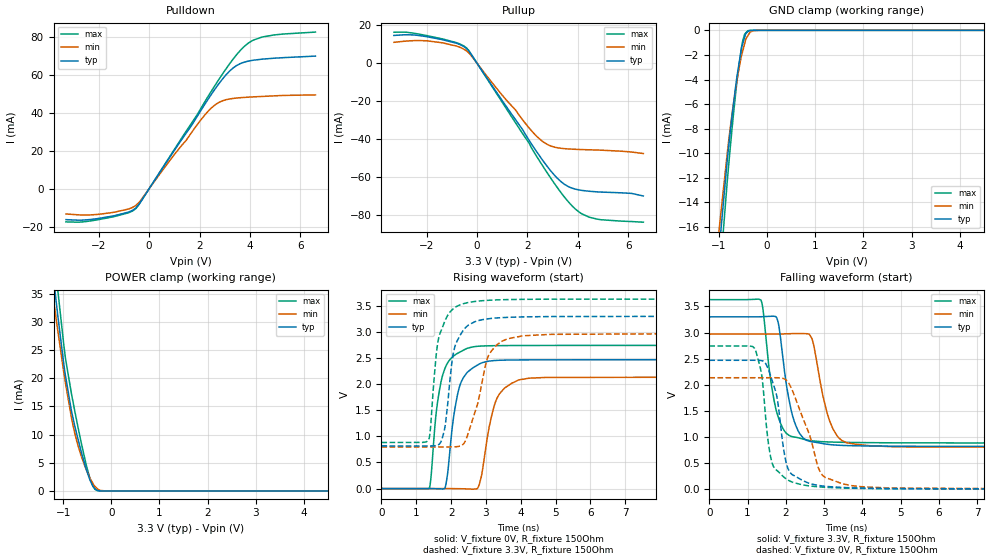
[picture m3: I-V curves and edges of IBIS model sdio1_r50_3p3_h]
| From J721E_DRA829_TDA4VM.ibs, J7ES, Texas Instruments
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|   r50_3p3_h
[Model]   sdio1_r50_3p3_h
Model_type   I/O
Polarity   Non-Inverting
Enable   Active-High
Vinl = 0
Vinh = 0.8
Vmeas = 1.65
Vref = 3.3
Cref = 2pF
Rref = 100000
|   typ   min   max
C_comp   2.899pF   2.635pF   3.167pF
[Voltage Range]   3.3   2.97   3.63
[Temperature Range]   27   150   -40
[Pullup Reference]   3.3   2.97   3.63
[Pulldown Reference]   0   0   0
[Power Clamp Reference]   3.3   2.97   3.63
[GND Clamp Reference]   0   0   0
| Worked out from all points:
|   slope of the pulldown table from 0 to 0.495 V, typ, clamps not added: 49.2 ohm
|   slope of the pullup table from 0 to 0.495 V, typ, clamps not added: 50.3 ohm
|   GND clamp passes 1 mA (typ) near -0.50 V on its own axis
|   POWER clamp passes 1 mA (typ) near -0.39 V on its own axis
|   falling waveform, V_fixture 3.3V, R_fixture 150Ohm: 20-80 % time 337ps typ, 401ps min, 323ps max; typ from 3.3 V to 0.817 V
|   rising waveform, V_fixture 0V, R_fixture 150Ohm: 20-80 % time 319ps typ, 386ps min, 306ps max; typ from 0 V to 2.47 V
|   rising waveform, V_fixture 3.3V, R_fixture 150Ohm: 20-80 % time 305ps typ, 492ps min, 309ps max; typ from 0.817 V to 3.3 V
|   falling waveform, V_fixture 0V, R_fixture 150Ohm: 20-80 % time 324ps typ, 574ps min, 258ps max; typ from 2.47 V to 0 V
[Pulldown]
|   Voltage   I(typ)   I(min)   I(max)
-3.3V     -16.37mA   -13.36mA   -17.55mA
-2.003V   -15.72mA   -13.55mA   -16.34mA
-825mV    -12.41mA   -10.77mA   -12.77mA
-528mV    -10.21mA   -8.836mA   -10.53mA
1.917V    38.43mA    33.99mA    39.31mA
2.363V    47.76mA    41.24mA    49.28mA
2.779V    55.67mA    45.65mA    57.95mA
3.184V    62.04mA    47.4mA     65.85mA
3.452V    64.93mA    47.89mA    70.52mA
3.937V    67.42mA    48.37mA    76.93mA
4.491V    68.47mA    48.75mA    80.18mA
6.6V      70.08mA    49.57mA    82.77mA
[GND Clamp]
|   Voltage   I(typ)   I(min)   I(max)
-3.3V     -160mA     -119.4mA   -217mA
-1.033V   -19.39mA   -17.52mA   -22.42mA
-825mV    -10.43mA   -9.877mA   -12.11mA
-716.1mV  -6.541mA   -6.437mA   -7.501mA
-627mV    -3.775mA   -4.073mA   -4.142mA
-537.9mV  -1.565mA   -2.149mA   -1.562mA
-508.2mV  -1.103mA   -1.7mA     -875.4uA
-468.6mV  -579.1uA   -1.102mA   -332.5uA
-399.3mV  -111.6uA   -431uA     -25.66uA
-349.8mV  -18.88uA   -131.7uA   -5.143uA
-171.6mV  -88.29nA   -2.802uA   -107.4nA
6.6V      0A         0A         0A
[Pullup]
|   Voltage   I(typ)   I(min)   I(max)
-3.3V     14.73mA    11.09mA    16.42mA
-1.993V   14.07mA    11.89mA    14.65mA
-825mV    10.65mA    9.143mA    10.95mA
-438.9mV  8.033mA    6.753mA    8.341mA
1.808V    -35.11mA   -29.93mA   -37.21mA
2.313V    -45.75mA   -37.91mA   -48.12mA
2.779V    -54.45mA   -42.85mA   -57.84mA
3.333V    -62.64mA   -44.97mA   -68.45mA
3.887V    -66.53mA   -45.51mA   -76.92mA
4.452V    -67.71mA   -45.77mA   -81.42mA
6.125V    -68.82mA   -46.93mA   -83.71mA
6.6V      -70.21mA   -47.75mA   -84.07mA
[POWER Clamp]
|   Voltage   I(typ)   I(min)   I(max)
-3.3V     224.5mA    191.3mA    262.6mA
-1.211V   38.57mA    34.7mA     44.22mA
-1.132V   32.63mA    29.7mA     37.31mA
-1.122V   31.9mA     29.08mA    36.46mA
-953.7mV  20.54mA    19.22mA    23.62mA
-825mV    14.09mA    12.89mA    17.14mA
-765.6mV  11.78mA    10.49mA    14.49mA
-636.9mV  7.356mA    6.549mA    9.056mA
-478.5mV  2.813mA    2.955mA    3.268mA
-399.3mV  1.162mA    1.587mA    1.168mA
-290.4mV  108.5uA    386.2uA    43.35uA
6.6V      0A         0A         0A
[Ramp]
R_load = 150
|   typ   min   max
dV/dt_r   1.48067/3.18947e-10   1.27987/3.85347e-10   1.64553/3.05434e-10
dV/dt_f   1.48934/3.37023e-10   1.30238/3.9807e-10   1.64759/3.22498e-10
[Falling Waveform]
V_fixture = 3.3V
V_fixture_min = 2.97V
V_fixture_max = 3.63V
R_fixture = 150Ohm
C_fixture = 0F
|   Time   V(typ)   V(min)   V(max)
0s        3.3V       2.969V     3.63V
1.345ns   3.302V     2.969V     3.624V
1.59ns    3.31V      2.969V     2.149V
1.79ns    3.217V     2.97V      1.403V
2.135ns   1.521V     2.978V     1.013V
2.36ns    1.064V     2.98V      976.9mV
2.675ns   908.1mV    2.892V     927.1mV
3.125ns   855.9mV    1.346V     904.3mV
3.585ns   835.3mV    890.5mV    896.3mV
10ns      817.4mV    798.6mV    883.7mV
[Rising Waveform]
V_fixture = 0V
V_fixture_min = 0V
V_fixture_max = 0V
R_fixture = 150Ohm
C_fixture = 0F
|   Time   V(typ)   V(min)   V(max)
0s        487.6uV    1.089mV    358.6uV
1.37ns    252.8uV    705.2uV    6.723mV
1.59ns    -2.491mV   527.8uV    1.55V
1.815ns   2.839mV    544.5uV    2.286V
2.175ns   1.768V     -1.302mV   2.586V
2.445ns   2.211V     -5.929mV   2.681V
2.81ns    2.386V     78.56mV    2.728V
3.325ns   2.456V     1.739V     2.738V
3.94ns    2.464V     2.08V      2.74V
10ns      2.468V     2.134V     2.743V
[Rising Waveform]
V_fixture = 3.3V
V_fixture_min = 2.97V
V_fixture_max = 3.63V
R_fixture = 150Ohm
C_fixture = 0F
|   Time   V(typ)   V(min)   V(max)
0s        817.4mV    798.6mV    883.7mV
1.35ns    817.3mV    798.4mV    928.3mV
1.645ns   843.4mV    798.3mV    2.889V
1.825ns   1.181V     798.3mV    3.215V
2.07ns    2.609V     799.1mV    3.448V
2.255ns   2.929V     814.4mV    3.519V
2.725ns   3.206V     1.544V     3.587V
3.06ns    3.251V     2.525V     3.606V
3.62ns    3.279V     2.868V     3.62V
10ns      3.3V       2.969V     3.63V
[Falling Waveform]
|Gnd
V_fixture = 0V
V_fixture_min = 0V
V_fixture_max = 0V
R_fixture = 150Ohm
C_fixture = 0F
|   Time   V(typ)   V(min)   V(max)
0s        2.468V     2.134V     2.743V
1.185ns   2.468V     2.134V     2.696V
1.37ns    2.461V     2.134V     2.174V
1.46ns    2.418V     2.134V     1.465V
1.645ns   2.07V      2.134V     489.8mV
1.995ns   545.3mV    2.097V     203.6mV
2.185ns   270.8mV    1.863V     130.6mV
2.9ns     66.87mV    324.9mV    42.65mV
3.475ns   33.01mV    103.6mV    22.79mV
10ns      486.9uV    1.089mV    358.5uV
